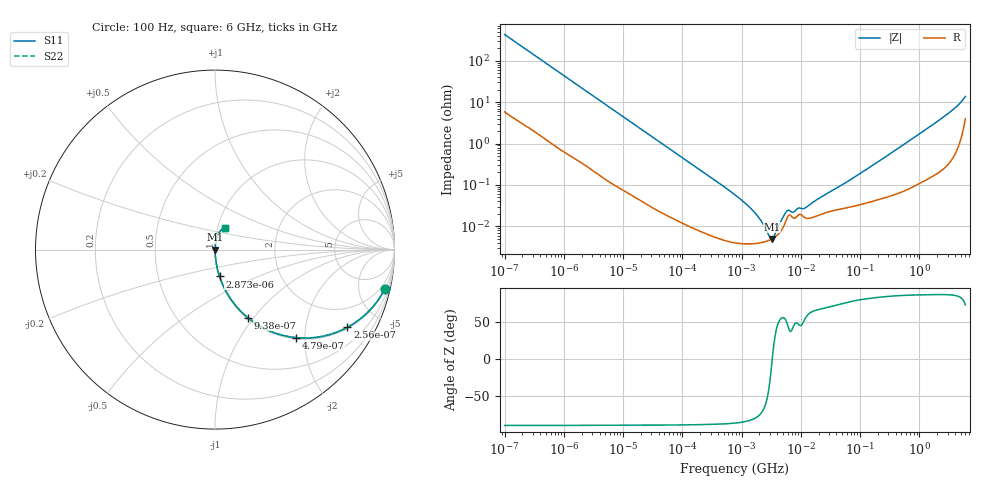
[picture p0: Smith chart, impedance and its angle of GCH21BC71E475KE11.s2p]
!Murata Part Number: GCH21BC71E475KE11
!These Parameters are Measured in Series Mode Connection
!Data Generated on Mar 13, 2026
!  o--ll--o
!Port1  Port2
!  o------o
!Operation Temp=25[degC], DC Bias Voltage=0[V]
!Freq. Start=100[Hz] Stop=6[GHz] 401[Steps]
# Hz S RI R 50
!Freq.(Hz) S11(Real) S11(Imag) S21(Real) S21(Imag) S12(Real) S12(Imag) S22(Real) S22(Imag)
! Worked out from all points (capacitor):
!   401 points, 100 Hz to 6 GHz, reference 50 ohm
!   read as one part in series: C = 3.7 uF near 109 Hz
!   lowest |Z| = 4.99 mohm at 3.246 MHz (marker M1)
!   series resonance near 3.294 MHz, so ESL is about 630 pH
!   S11 on the Smith chart (normalised r, x): 100 Hz: 1.12, -8.58; 256 Hz: 1.05, -3.38; 479 Hz: 1.03, -1.82; 938 Hz: 1.01, -0.93; 2.873 kHz: 1.00, -0.31; 6 GHz: 1.08, +0.26
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100  0.9458 -0.2197  0.0542 0.2197  0.0542 0.2197  0.9458 -0.2197
164  0.8706 -0.3289  0.1294 0.3289  0.1294 0.3289  0.8706 -0.3289
256  0.7375 -0.433  0.2625 0.433  0.2625 0.433  0.7375 -0.433
479  0.4526 -0.4907  0.5474 0.4907  0.5474 0.4907  0.4526 -0.4907
938  0.1822 -0.379  0.8178 0.379  0.8178 0.379  0.1822 -0.379
2008  0.0489 -0.208  0.9511 0.208  0.9511 0.208  0.0489 -0.208
2873  0.0254 -0.1497  0.9746 0.1497  0.9746 0.1497  0.0254 -0.1497
8416  0.00366 -0.0528  0.9963 0.0528  0.9963 0.0528  0.00366 -0.0528
40335  0.000357 -0.0113  0.9996 0.0113  0.9996 0.0113  0.000357 -0.0113
774597  4.02e-05 -0.000575  1 0.000575  1 0.000575  4.02e-05 -0.000575
1516199  3.8e-05 -0.000247  1 0.000247  1 0.000247  3.8e-05 -0.000247
2481164  4.26e-05 -8.4e-05  1 8.4e-05  1 8.4e-05  4.26e-05 -8.4e-05
3245845  4.97e-05 -4.3e-06  1 4.3e-06  1 4.3e-06  4.97e-05 -4.3e-06
4246196  6.65e-05 7.96e-05  0.9999 -7.96e-05  0.9999 -7.96e-05  6.65e-05 7.96e-05
5554849  0.000131 0.000171  0.9999 -0.000171  0.9999 -0.000171  0.000131 0.000171
6075234  0.000177 0.000171  0.9998 -0.000171  0.9998 -0.000171  0.000177 0.000171
7266822  0.000163 0.000144  0.9998 -0.000144  0.9998 -0.000144  0.000163 0.000144
1.137099e7  0.000166 0.000212  0.9998 -0.000212  0.9998 -0.000212  0.000166 0.000212
1.555665e7  0.000163 0.000332  0.9998 -0.000332  0.9998 -0.000332  0.000163 0.000332
3.124326e8  0.000559 0.00548  0.9994 -0.00548  0.9994 -0.00548  0.000559 0.00548
2.679998e9  0.00464 0.0455  0.9954 -0.0455  0.9954 -0.0455  0.00464 0.0455
6e9  0.0535 0.1192  0.9465 -0.1192  0.9465 -0.1192  0.0535 0.1192
